| IBIS file stm32u3b5_3c5_wlcsp72_smps.ibs
[IBIS ver] 4.2
[File name] stm32u3b5_3c5_wlcsp72_smps.ibs
[File Rev] 0.1
[Date] 09-03-2026
[Source] Data Created at STMicroelectronics
[Notes]  File originated from ELDO simulations.
[Disclaimer]  This information is for modeling purpose only and is
   not guaranted. The information is subject to change without
   notice.
[Copyright] Copyright 2026 STMicroelectronics Inc.
|   Component stm32u3b5_3c5_wlcsp72_smps
[Component] stm32u3b5_3c5_wlcsp72_smps
[Manufacturer] STMicroelectronics
[Package]
| variable   typ   min   max
R_pkg  0  NA  NA
L_pkg  0  NA  NA
C_pkg  0  NA  NA
[Pin]   signal_name   model_name
A1  VDD  power
A3  VDDUSB  power
A5  PC12  io8_ft_100m_hslv
A7  PD2  io8_ft_100m_hslv
A9  PB3  io8_ft_100m_hslv
A11  PB7  io8_ft_100m_hslv
A13  VSS  gnd
A15  VDD  power
B2  VSS  gnd
B4  PC10  io8_ft_100m_hslv
B6  PC11  io8_ft_100m_hslv
B8  PB4  io8_ft_100m_hslv
B10  PB8  io8_ft_100m_hslv
B12  PB9  io8_ft_100m_hslv
B14  PC13  io8_ft_100m_v33
B16  VBAT  power
C1  PA11  io8usb_ft_phy
C3  PA12  io8usb_ft_phy
C5  PA13  io8_ft_100m
C7  PA14  io8_ft_100m
C9  PB5  io8_ft_100m_hslv
C11  PH3-BOOT0  io8_ft_100m_hslv
C13  PC15-OSC32_OUT  io_ft_tamp
C15  PC14-OSC32_IN  io_ft_tamp
D2  PA8  io8_ft_100m_hslv
D4  PA9  io8_ft_100m
D6  PA10  io8_ft_100m
D8  PA15  io8_ft_100m
D10  PB6  io8_ft_100m_hslv
D12  PC1  io8_ft_100m_hslv
D14  PH1-OSC_OUT  io8_ft_100m
D16  PH0-OSC_IN  io8_ft_100m
E1  PC7  io8_ft_100m_hslv
E3  PC6  io8_ft_100m_hslv
E5  PC8  io8_ft_100m_hslv
E7  PC9  io8_ft_100m_hslv
E9  PA1  io8_ft_100m_hslv
E11  PC2  io8_ft_100m_hslv
E13  PC3  io8_ft_100m_hslv
E15  PC0  io8_ft_100m_hslv
F2  PB13  io8_ft_100m_hslv
F4  PB14  io8_ft_100m_hslv
F6  PE14  io8_ft_100m_hslv
F8  PE13  io8_ft_100m_hslv
F10  PA7  io8_ft_100m_hslv
F12  PA4  io8_ft_100m_hslv
F14  PA0  io8_ft_100m
F16  NRST  ioreset_v33
G1  PB15  io8_ft_100m
G3  PB10  io8_ft_100m_hslv
G5  PB11  io8_ft_100m_hslv
G7  PE10  io8_ft_100m_hslv
G9  PB0  io8_ft_100m_hslv
G11  PA5  io8_ft_100m
G13  PA2  io8_ft_100m_hslv
G15  VSSA_VREFM  nc
H2  VDD  power
H4  VSS  gnd
H6  VSSSMPS  nc
H8  PE11  io8_ft_100m_hslv
H10  PB2  io8_ft_100m_hslv
H12  PA6  io8_ft_100m_hslv
H14  PA3  io8_ft_100m_hslv
H16  VDDA_VREFP  nc
J1  PB12  io8_ft_100m_hslv
J3  VDD11  nc
J5  VDDSMPS  nc
J7  VLXSMPS  nc
J9  PE12  io8_ft_100m_hslv
J11  PB1  io8_ft_100m_hslv
J13  VDD  power
J15  VSS  gnd
[Package Model]   42a-wlcsp-72-260114
[Pin Mapping]   pulldown_ref   pullup_ref   | Comment
A1  nc  vddio
A3  nc  vddusb
A5  gndio  vddio
A7  gndio  vddio
A9  gndio  vddio
A11  gndio  vddio
A13  gndio  nc
A15  nc  vddio
B2  gndio  nc
B4  gndio  vddio
B6  gndio  vddio
B8  gndio  vddio
B10  gndio  vddio
B12  gndio  vddio
B14  gndio  vsw
B16  nc  vsw
C1  gndio  vddusb  | Depending on IO usage
| C1  gndio  vddio  | Depending on IO usage
C3  gndio  vddusb  | Depending on IO usage
| C3  gndio  vddio  | Depending on IO usage
C5  gndio  vddio
C7  gndio  vddio
C9  gndio  vddio
C11  gndio  vddio
C13  gndio  vsw
C15  gndio  vsw
D2  gndio  vddio
D4  gndio  vddio
D6  gndio  vddio
D8  gndio  vddio
D10  gndio  vddio
D12  gndio  vddio
D14  gndio  vddio
D16  gndio  vddio
E1  gndio  vddio
E3  gndio  vddio
E5  gndio  vddio
E7  gndio  vddio
E9  gndio  vddio
E11  gndio  vddio
E13  gndio  vddio
E15  gndio  vddio
F2  gndio  vddio
F4  gndio  vddio
F6  gndio  vddio
F8  gndio  vddio
F10  gndio  vddio
F12  gndio  vddio
F14  gndio  vddio
F16  gndio  vddio
G1  gndio  vddio
G3  gndio  vddio
G5  gndio  vddio
G7  gndio  vddio
G9  gndio  vddio
G11  gndio  vddio
G13  gndio  vddio
G15  nc  nc
H2  nc  vddio
H4  gndio  nc
H6  nc  nc
H8  gndio  vddio
H10  gndio  vddio
H12  gndio  vddio
H14  gndio  vddio
H16  nc  nc
J1  gndio  vddio
J3  nc  nc
J5  nc  nc
J7  nc  nc
J9  gndio  vddio
J11  gndio  vddio
J13  nc  vddio
J15  gndio  nc
|[Diff Pin]  inv_pin  vdiff  tdelay_typ  tdelay_min  tdelay_max
|C3  C1  NA  NA  NA  NA
[Model Selector] io8_ft_100m
io8_ft_100m_ls_1v2  "GPIO 100MHz - 5V tolerant - low speed - 1.2V range"
io8_ft_100m_ls_1v8  "GPIO 100MHz - 5V tolerant - low speed - 1.8V range"
io8_ft_100m_ls_3v3  "GPIO 100MHz - 5V tolerant - low speed - 3.3V range"
io8_ft_100m_ms_1v2  "GPIO 100MHz - 5V tolerant - med speed - 1.2V range"
io8_ft_100m_ms_1v8  "GPIO 100MHz - 5V tolerant - med speed - 1.8V range"
io8_ft_100m_ms_3v3  "GPIO 100MHz - 5V tolerant - med speed - 3.3V range"
io8_ft_100m_fs_1v2  "GPIO 100MHz - 5V tolerant - fast speed - 1.2V range"
io8_ft_100m_fs_1v8  "GPIO 100MHz - 5V tolerant - fast speed - 1.8V range"
io8_ft_100m_fs_3v3  "GPIO 100MHz - 5V tolerant - fast speed - 3.3V range"
io8_ft_100m_hs_1v2  "GPIO 100MHz - 5V tolerant - high speed - 1.2V range"
io8_ft_100m_hs_1v8  "GPIO 100MHz - 5V tolerant - high speed - 1.8V range"
io8_ft_100m_hs_3v3  "GPIO 100MHz - 5V tolerant - high speed - 3.3V range"
[Model Selector] io8_ft_100m_hslv
io8_ft_100m_ls_1v2  "GPIO 100MHz - 5V tolerant - low speed - 1.2V range"
io8_ft_100m_ls_1v8  "GPIO 100MHz - 5V tolerant - low speed - 1.8V range"
io8_ft_100m_ls_3v3  "GPIO 100MHz - 5V tolerant - low speed - 3.3V range"
io8_ft_100m_ms_1v2  "GPIO 100MHz - 5V tolerant - med speed - 1.2V range"
io8_ft_100m_ms_1v8  "GPIO 100MHz - 5V tolerant - med speed - 1.8V range"
io8_ft_100m_ms_3v3  "GPIO 100MHz - 5V tolerant - med speed - 3.3V range"
io8_ft_100m_fs_1v2  "GPIO 100MHz - 5V tolerant - fast speed - 1.2V range"
io8_ft_100m_fs_1v8  "GPIO 100MHz - 5V tolerant - fast speed - 1.8V range"
io8_ft_100m_fs_3v3  "GPIO 100MHz - 5V tolerant - fast speed - 3.3V range"
io8_ft_100m_hs_1v2  "GPIO 100MHz - 5V tolerant - high speed - 1.2V range"
io8_ft_100m_hs_1v8  "GPIO 100MHz - 5V tolerant - high speed - 1.8V range"
io8_ft_100m_hs_3v3  "GPIO 100MHz - 5V tolerant - high speed - 3.3V range"
io8_ft_100m_hslv_ls_1v2  "GPIO 100MHz low voltage optimization - 5V tolerant - low speed - 1.2V range"
io8_ft_100m_hslv_ls_1v8  "GPIO 100MHz low voltage optimization - 5V tolerant - low speed - 1.8V range"
io8_ft_100m_hslv_ls_2v5  "GPIO 100MHz low voltage optimization - 5V tolerant - low speed - 3.3V range"
io8_ft_100m_hslv_ms_1v2  "GPIO 100MHz low voltage optimization - 5V tolerant - med speed - 1.2V range"
io8_ft_100m_hslv_ms_1v8  "GPIO 100MHz low voltage optimization - 5V tolerant - med speed - 1.8V range"
io8_ft_100m_hslv_ms_2v5  "GPIO 100MHz low voltage optimization - 5V tolerant - med speed - 3.3V range"
io8_ft_100m_hslv_fs_1v2  "GPIO 100MHz low voltage optimization - 5V tolerant - fast speed - 1.2V range"
io8_ft_100m_hslv_fs_1v8  "GPIO 100MHz low voltage optimization - 5V tolerant - fast speed - 1.8V range"
io8_ft_100m_hslv_fs_2v5  "GPIO 100MHz low voltage optimization - 5V tolerant - fast speed - 3.3V range"
io8_ft_100m_hslv_hs_1v2  "GPIO 100MHz low voltage optimization - 5V tolerant - high speed - 1.2V range"
io8_ft_100m_hslv_hs_1v8  "GPIO 100MHz low voltage optimization - 5V tolerant - high speed - 1.8V range"
io8_ft_100m_hslv_hs_2v5  "GPIO 100MHz low voltage optimization - 5V tolerant - high speed - 3.3V range"
[Model Selector] io8_ft_100m_v33
io8_ft_100m_v33_ls_1v2  "GPIO_V33 100MHz - 5V tolerant - low speed - 1.2V range"
io8_ft_100m_v33_ls_1v8  "GPIO_V33 100MHz - 5V tolerant - low speed - 1.8V range"
io8_ft_100m_v33_ls_3v3  "GPIO_V33 100MHz - 5V tolerant - low speed - 3.3V range"
io8_ft_100m_v33_ms_1v2  "GPIO_V33 100MHz - 5V tolerant - med speed - 1.2V range"
io8_ft_100m_v33_ms_1v8  "GPIO_V33 100MHz - 5V tolerant - med speed - 1.8V range"
io8_ft_100m_v33_ms_3v3  "GPIO_V33 100MHz - 5V tolerant - med speed - 3.3V range"
io8_ft_100m_v33_fs_1v2  "GPIO_V33 100MHz - 5V tolerant - fast speed - 1.2V range"
io8_ft_100m_v33_fs_1v8  "GPIO_V33 100MHz - 5V tolerant - fast speed - 1.8V range"
io8_ft_100m_v33_fs_3v3  "GPIO_V33 100MHz - 5V tolerant - fast speed - 3.3V range"
io8_ft_100m_v33_hs_1v2  "GPIO_V33 100MHz - 5V tolerant - high speed - 1.2V range"
io8_ft_100m_v33_hs_1v8  "GPIO_V33 100MHz - 5V tolerant - high speed - 1.8V range"
io8_ft_100m_v33_hs_3v3  "GPIO_V33 100MHz - 5V tolerant - high speed - 3.3V range"
[Model Selector] io8usb_ft_phy
io8_ft_100m_ls_1v2  "GPIO 100MHz - 5V tolerant - low speed - 1.2V range"
io8_ft_100m_ls_1v8  "GPIO 100MHz - 5V tolerant - low speed - 1.8V range"
io8_ft_100m_ls_3v3  "GPIO 100MHz - 5V tolerant - low speed - 3.3V range"
io8_ft_100m_ms_1v2  "GPIO 100MHz - 5V tolerant - med speed - 1.2V range"
io8_ft_100m_ms_1v8  "GPIO 100MHz - 5V tolerant - med speed - 1.8V range"
io8_ft_100m_ms_3v3  "GPIO 100MHz - 5V tolerant - med speed - 3.3V range"
io8_ft_100m_fs_1v2  "GPIO 100MHz - 5V tolerant - fast speed - 1.2V range"
io8_ft_100m_fs_1v8  "GPIO 100MHz - 5V tolerant - fast speed - 1.8V range"
io8_ft_100m_fs_3v3  "GPIO 100MHz - 5V tolerant - fast speed - 3.3V range"
io8_ft_100m_hs_1v2  "GPIO 100MHz - 5V tolerant - high speed - 1.2V range"
io8_ft_100m_hs_1v8  "GPIO 100MHz - 5V tolerant - high speed - 1.8V range"
io8_ft_100m_hs_3v3  "GPIO 100MHz - 5V tolerant - high speed - 3.3V range"
io8usb_ft_phy_hs_3v3   "USB full speed"
io8usb_ft_phy_ls_3v3   "USB low speed"
[Model Selector] io_ft_tamp
io_ft_tamp_ls_1v2 "io8_ft tamp low speed @ 1.2V"
io_ft_tamp_ls_1v8 "io8_ft tamp low speed @ 1.8V"
io_ft_tamp_ls_3v3 "io8_ft tamp low speed @ 3.3V"
io_ft_tamp_ms_1v2 "io8_ft tamp med speed @ 1.2V"
io_ft_tamp_ms_1v8 "io8_ft tamp med speed @ 1.8V"
io_ft_tamp_ms_3v3 "io8_ft tamp med speed @ 3.3V"
io_ft_tamp_fs_1v2 "io8_ft tamp fast speed @ 1.2V"
io_ft_tamp_fs_1v8 "io8_ft tamp fast speed @ 1.8V"
io_ft_tamp_fs_3v3 "io8_ft tamp fast speed @ 3.3V"
io_ft_tamp_hs_1v2 "io8_ft tamp high speed @ 1.2V"
io_ft_tamp_hs_1v8 "io8_ft tamp high speed @ 1.8V"
io_ft_tamp_hs_3v3 "io8_ft tamp high speed @ 3.3V"
[Model Selector] ioreset_v33
ioreset_v33_1v2 "Reset PAD. 5V tolerant. 1.2V range"
ioreset_v33_1v8 "Reset PAD. 5V tolerant. 1.8V range"
ioreset_v33_3v3 "Reset PAD. 5V tolerant. 3.3V range"
[Define Package Model]  42a-wlcsp-72-260114
[Manufacturer]  Unknown
[OEM]  Unknown
[Description]  None
[Number Of Pins]  70
[Pin Numbers]
| Pin Num   Terminal Name
F16 | NRST
F14 | PA0
E9 | PA1
G13 | PA2
H14 | PA3
F12 | PA4
G11 | PA5
H12 | PA6
F10 | PA7
D2 | PA8
D4 | PA9
D6 | PA10
C1 | PA11
C3 | PA12
C5 | PA13
C7 | PA14
D8 | PA15
G9 | PB0
J11 | PB1
H10 | PB2
A9 | PB3
B8 | PB4
C9 | PB5
D10 | PB6
A11 | PB7
B10 | PB8
B12 | PB9
G3 | PB10
G5 | PB11
J1 | PB12
F2 | PB13
F4 | PB14
G1 | PB15
E15 | PC0
D12 | PC1
E11 | PC2
E13 | PC3
E3 | PC6
E1 | PC7
E5 | PC8
E7 | PC9
B4 | PC10
B6 | PC11
A5 | PC12
B14 | PC13
C15 | PC14-OSC32_IN
C13 | PC15-OSC32_OUT
A7 | PD2
G7 | PE10
H8 | PE11
J9 | PE12
F8 | PE13
F6 | PE14
D16 | PH0-OSC_IN
D14 | PH1-OSC_OUT
C11 | PH3-BOOT0
J3 | VDD11
B16 | VBAT
A1 | VDD
A15 | VDD
H2 | VDD
H16 | VDDA_VREFP
J5 | VDDSMPS
A3 | VDDUSB
J7 | VLXSMPS
A13 | VSS
H4 | VSS
J15 | VSS
G15 | VSSA_VREFM
H6 | VSSSMPS
|[Merged Pins]  H2
|J13  |  VDD
|[Merged Pins]  A13
|B2  |  VSS
[Model Data]
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[End Model Data]
[End Package Model]
|End [Component]
| Models and submodels in the file (53): io8_ft_100m_fs_1v2 (I/O), io8_ft_100m_fs_1v8 (I/O), io8_ft_100m_fs_3v3 (I/O), io8_ft_100m_hs_1v2 (I/O), io8_ft_100m_hs_1v8 (I/O), io8_ft_100m_hs_3v3 (I/O), io8_ft_100m_hslv_fs_1v2 (I/O), io8_ft_100m_hslv_fs_1v8 (I/O), io8_ft_100m_hslv_fs_2v5 (I/O), io8_ft_100m_hslv_hs_1v2 (I/O), io8_ft_100m_hslv_hs_1v8 (I/O), io8_ft_100m_hslv_hs_2v5 (I/O), io8_ft_100m_hslv_ls_1v2 (I/O), io8_ft_100m_hslv_ls_1v8 (I/O), io8_ft_100m_hslv_ls_2v5 (I/O), io8_ft_100m_hslv_ms_1v2 (I/O), io8_ft_100m_hslv_ms_1v8 (I/O), io8_ft_100m_hslv_ms_2v5 (I/O), io8_ft_100m_ls_1v2 (I/O), io8_ft_100m_ls_1v8 (I/O), io8_ft_100m_ls_3v3 (I/O), io8_ft_100m_ms_1v2 (I/O), io8_ft_100m_ms_1v8 (I/O), io8_ft_100m_ms_3v3 (I/O), io8_ft_100m_v33_fs_1v2 (I/O), io8_ft_100m_v33_fs_1v8 (I/O), io8_ft_100m_v33_fs_3v3 (I/O), io8_ft_100m_v33_hs_1v2 (I/O), io8_ft_100m_v33_hs_1v8 (I/O), io8_ft_100m_v33_hs_3v3 (I/O), io8_ft_100m_v33_ls_1v2 (I/O), io8_ft_100m_v33_ls_1v8 (I/O), io8_ft_100m_v33_ls_3v3 (I/O), io8_ft_100m_v33_ms_1v2 (I/O), io8_ft_100m_v33_ms_1v8 (I/O), io8_ft_100m_v33_ms_3v3 (I/O), io8usb_ft_phy_hs_3v3 (I/O), io8usb_ft_phy_ls_3v3 (I/O), io_ft_tamp_fs_1v2 (I/O), io_ft_tamp_fs_1v8 (I/O), io_ft_tamp_fs_3v3 (I/O), io_ft_tamp_hs_1v2 (I/O), io_ft_tamp_hs_1v8 (I/O), io_ft_tamp_hs_3v3 (I/O), io_ft_tamp_ls_1v2 (I/O), io_ft_tamp_ls_1v8 (I/O), io_ft_tamp_ls_3v3 (I/O), io_ft_tamp_ms_1v2 (I/O), io_ft_tamp_ms_1v8 (I/O), io_ft_tamp_ms_3v3 (I/O), ioreset_v33_1v2 (I/O_open_drain), ioreset_v33_1v8 (I/O_open_drain), ioreset_v33_3v3 (I/O_open_drain)
